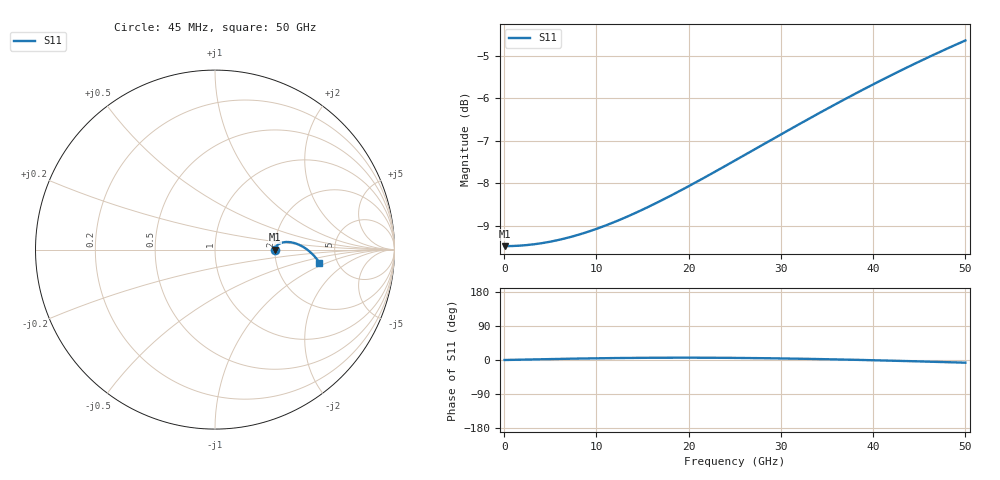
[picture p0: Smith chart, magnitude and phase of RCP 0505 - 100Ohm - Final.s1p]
!Vishay Electro-Films Inc.
!RCP Family
!Case Size 0505
!Assembly Style Surface Mount
!11/2/2015
!efi@vishay.com
# GHz S MA R 50
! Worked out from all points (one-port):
!   801 points, 45 MHz to 50 GHz, reference 50 ohm
!   lowest |S11| = -9.5 dB at 45 MHz (marker M1), VSWR 2.01, Z = 100 + j0.0305 ohm
!   |S11| at or under -10 dB: nowhere
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0.045  0.3355 0.0
1.54365  0.3359 0.8
3.104744  0.3371 1.6
4.665838  0.3391 2.3
6.289375  0.342 3.1
7.788025  0.3454 3.7
9.286675  0.3495 4.3
10.84777  0.3544 4.8
12.53375  0.3604 5.3
15.59349  0.3731 5.9
18.77812  0.3884 6.1
21.96276  0.4056 6.0
25.0225  0.4233 5.5
28.14469  0.4425 4.8
29.70578  0.4524 4.3
31.26687  0.4625 3.7
32.82797  0.4727 3.0
34.38906  0.483 2.4
35.95016  0.4933 1.6
37.51125  0.5038 0.8
39.07234  0.5142 -0.1
40.63344  0.5246 -1.0
42.19453  0.535 -1.9
43.75563  0.5454 -2.9
46.50315  0.5635 -4.7
49.0009  0.5798 -6.4
49.75023  0.5846 -6.9
50  0.5862 -7.1
